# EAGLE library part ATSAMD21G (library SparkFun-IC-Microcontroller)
Atmel SAMD21G SMART ARM-Based Microcontroller The Atmel ® | SMART ™ SAM D21 is a series of low-power microcontrollers using the 32-bit ARM ® Cortex ® -M0+ processor, and ranging from 32- to 64-pins with up to 256KB Flash and 32KB of SRAM. The SAM D21 devices operate at a maximum frequency of 48MHz and reach 2.46 CoreMark/MHz. They are designed for simple and intuitive migration with identical peripheral modules, hex compatible code, identical linear address map and pin compatible migration paths between all devices in the product series. All devices include intelligent and flexible peripherals, Atmel Event System for inter-peripheral signaling, and support for capacitive touch button, slider and wheel user interfaces. Datasheet SparkFun Products SparkFun SAMD21 Mini Breakout (DEV-13664) SparkFun SAMD21 Dev Breakout (DEV-13672) (DEV-14926)
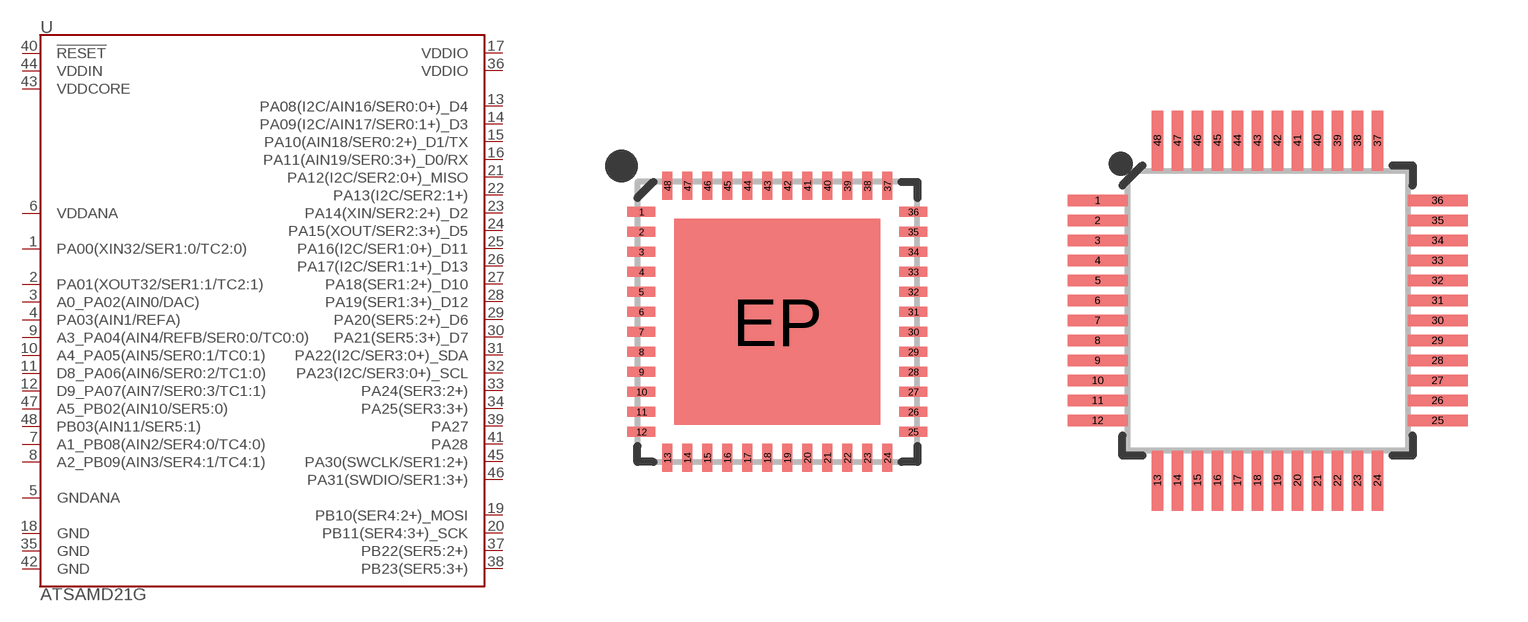
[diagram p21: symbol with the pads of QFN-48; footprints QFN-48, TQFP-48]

Designator prefix U

## ATSAMD21G-M (PROD_ID: IC-13064)  [QFN-48]
1  PA00(XIN32/SER1:0/TC2:0)
2  PA01(XOUT32/SER1:1/TC2:1)
3  A0_PA02(AIN0/DAC)
4  PA03(AIN1/REFA)
5  GNDANA
6  VDDANA
7  A1_PB08(AIN2/SER4:0/TC4:0)
8  A2_PB09(AIN3/SER4:1/TC4:1)
9  A3_PA04(AIN4/REFB/SER0:0/TC0:0)
10  A4_PA05(AIN5/SER0:1/TC0:1)
11  D8_PA06(AIN6/SER0:2/TC1:0)
12  D9_PA07(AIN7/SER0:3/TC1:1)
13  PA08(I2C/AIN16/SER0:0+)_D4
14  PA09(I2C/AIN17/SER0:1+)_D3
15  PA10(AIN18/SER0:2+)_D1/TX
16  PA11(AIN19/SER0:3+)_D0/RX
17  VDDIO
18  GND
19  PB10(SER4:2+)_MOSI
20  PB11(SER4:3+)_SCK
21  PA12(I2C/SER2:0+)_MISO
22  PA13(I2C/SER2:1+)
23  PA14(XIN/SER2:2+)_D2
24  PA15(XOUT/SER2:3+)_D5
25  PA16(I2C/SER1:0+)_D11
26  PA17(I2C/SER1:1+)_D13
27  PA18(SER1:2+)_D10
28  PA19(SER1:3+)_D12
29  PA20(SER5:2+)_D6
30  PA21(SER5:3+)_D7
31  PA22(I2C/SER3:0+)_SDA
32  PA23(I2C/SER3:0+)_SCL
33  PA24(SER3:2+)
34  PA25(SER3:3+)
35  GND
36  VDDIO
37  PB22(SER5:2+)
38  PB23(SER5:3+)
39  PA27
40  !RESET!
41  PA28
42  GND
43  VDDCORE
44  VDDIN
45  PA30(SWCLK/SER1:2+)
46  PA31(SWDIO/SER1:3+)
47  A5_PB02(AIN10/SER5:0)
48  PB03(AIN11/SER5:1)

## ATSAMD21G-A (PROD_ID: IC-13064)  [TQFP-48]
Pads as for QFN-48

## ATSAMD21G (PROD_ID: IC-14066)  [QFN-48_NO_EXPOSED_PAD]
Pads as for QFN-48

## Footprint QFN-48 (pad centres in mm)
48-pin QFN (7x7mm, 0.5mm pitch) Used on: ATSAMD21G
smd 0.7 x 0.25: 1 -3.4,2.75; 2 -3.4,2.25; 3 -3.4,1.75; 4 -3.4,1.25; 5 -3.4,0.75; 6 -3.4,0.25; 7 -3.4,-0.25; 8 -3.4,-0.75; 9 -3.4,-1.25; 10 -3.4,-1.75; 11 -3.4,-2.25; 12 -3.4,-2.75; 25 3.4,-2.75; 26 3.4,-2.25; 27 3.4,-1.75; 28 3.4,-1.25; 29 3.4,-0.75; 30 3.4,-0.25; 31 3.4,0.25; 32 3.4,0.75; 33 3.4,1.25; 34 3.4,1.75; 35 3.4,2.25; 36 3.4,2.75
smd 0.25 x 0.7: 13 -2.75,-3.4; 14 -2.25,-3.4; 15 -1.75,-3.4; 16 -1.25,-3.4; 17 -0.75,-3.4; 18 -0.25,-3.4; 19 0.25,-3.4; 20 0.75,-3.4; 21 1.25,-3.4; 22 1.75,-3.4; 23 2.25,-3.4; 24 2.75,-3.4; 37 2.75,3.4; 38 2.25,3.4; 39 1.75,3.4; 40 1.25,3.4; 41 0.75,3.4; 42 0.25,3.4; 43 -0.25,3.4; 44 -0.75,3.4; 45 -1.25,3.4; 46 -1.75,3.4; 47 -2.25,3.4; 48 -2.75,3.4
smd 5.15 x 5.15: EP 0,0

## Footprint TQFP-48 (pad centres in mm)
48-pin TQFP (7x7mm, 0.5mm pitch) Used on: ATSAMD21G
smd 1.5 x 0.28: 1 -4.25,2.75; 2 -4.25,2.25; 3 -4.25,1.75; 4 -4.25,1.25; 5 -4.25,0.75; 6 -4.25,0.25; 7 -4.25,-0.25; 8 -4.25,-0.75; 9 -4.25,-1.25; 10 -4.25,-1.75; 11 -4.25,-2.25; 12 -4.25,-2.75; 25 4.25,-2.75; 26 4.25,-2.25; 27 4.25,-1.75; 28 4.25,-1.25; 29 4.25,-0.75; 30 4.25,-0.25; 31 4.25,0.25; 32 4.25,0.75; 33 4.25,1.25; 34 4.25,1.75; 35 4.25,2.25; 36 4.25,2.75
smd 0.28 x 1.5: 13 -2.75,-4.25; 14 -2.25,-4.25; 15 -1.75,-4.25; 16 -1.25,-4.25; 17 -0.75,-4.25; 18 -0.25,-4.25; 19 0.25,-4.25; 20 0.75,-4.25; 21 1.25,-4.25; 22 1.75,-4.25; 23 2.25,-4.25; 24 2.75,-4.25; 37 2.75,4.25; 38 2.25,4.25; 39 1.75,4.25; 40 1.25,4.25; 41 0.75,4.25; 42 0.25,4.25; 43 -0.25,4.25; 44 -0.75,4.25; 45 -1.25,4.25; 46 -1.75,4.25; 47 -2.25,4.25; 48 -2.75,4.25

## Footprint QFN-48_NO_EXPOSED_PAD (pad centres in mm)
48-pin QFN (7x7mm, 0.5mm pitch) This package is used with the SAMD21 and has had the no-connect-exposed-pad underneath removed for situations that require tight routing. Use at your own risk!.</p
smd 0.7 x 0.25: 1 -3.4,2.75; 2 -3.4,2.25; 3 -3.4,1.75; 4 -3.4,1.25; 5 -3.4,0.75; 6 -3.4,0.25; 7 -3.4,-0.25; 8 -3.4,-0.75; 9 -3.4,-1.25; 10 -3.4,-1.75; 11 -3.4,-2.25; 12 -3.4,-2.75; 25 3.4,-2.75; 26 3.4,-2.25; 27 3.4,-1.75; 28 3.4,-1.25; 29 3.4,-0.75; 30 3.4,-0.25; 31 3.4,0.25; 32 3.4,0.75; 33 3.4,1.25; 34 3.4,1.75; 35 3.4,2.25; 36 3.4,2.75
smd 0.25 x 0.7: 13 -2.75,-3.4; 14 -2.25,-3.4; 15 -1.75,-3.4; 16 -1.25,-3.4; 17 -0.75,-3.4; 18 -0.25,-3.4; 19 0.25,-3.4; 20 0.75,-3.4; 21 1.25,-3.4; 22 1.75,-3.4; 23 2.25,-3.4; 24 2.75,-3.4; 37 2.75,3.4; 38 2.25,3.4; 39 1.75,3.4; 40 1.25,3.4; 41 0.75,3.4; 42 0.25,3.4; 43 -0.25,3.4; 44 -0.75,3.4; 45 -1.25,3.4; 46 -1.75,3.4; 47 -2.25,3.4; 48 -2.75,3.4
